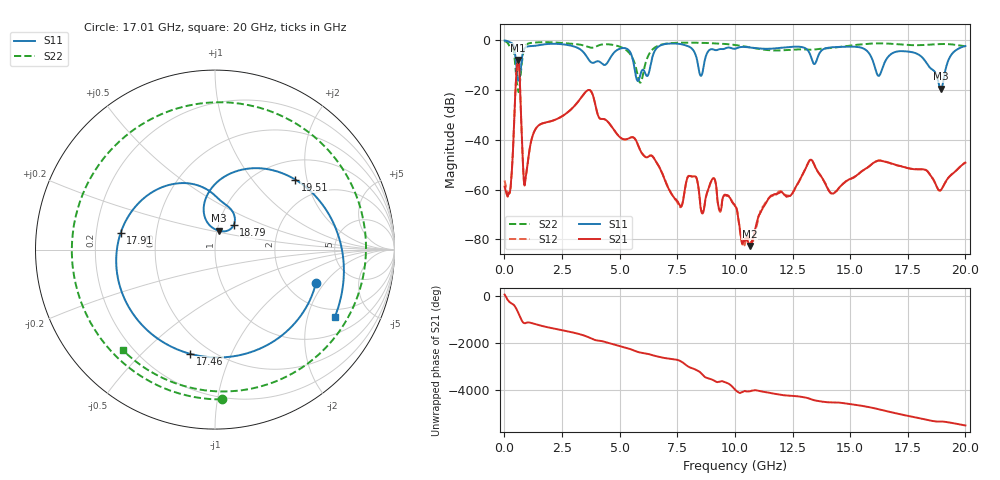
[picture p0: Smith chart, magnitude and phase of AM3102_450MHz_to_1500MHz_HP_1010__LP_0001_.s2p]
!Agilent Technologies,E8364B,MY43040894,A.07.50.67
!Agilent E8364B: A.07.50.67
!Date: Thursday, January 11, 2018 06:09:56
!Correction: S11(Full 2 Port(1,2))
!S21(Full 2 Port(1,2))
!S12(Full 2 Port(1,2))
!S22(Full 2 Port(1,2))
!S2P File: Measurements: S11, S21, S12, S22:
# Hz S  dB  R 50
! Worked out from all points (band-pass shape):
!   1601 points, 10 MHz to 20 GHz, reference 50 ohm
!   highest |S21| = -7.89 dB at 597.2 MHz (marker M1); lowest = -82.7 dB at 10.64 GHz (marker M2)
!   |S21| within 3 dB of the highest: 543 MHz to 644.9 MHz (101.9 MHz wide, 17.2 % of centre)
!   lowest |S11| = -19.4 dB at 18.94 GHz (marker M3), VSWR 1.24, Z = 51.1 + j10.8 ohm
!   |S11| at or under -10 dB: 5.621 GHz to 6.343 GHz (721.7 MHz wide, 12.1 % of centre); 16.05 GHz to 16.45 GHz (400.1 MHz wide, 2.46 % of centre); 18.38 GHz to 19.19 GHz (811.5 MHz wide, 4.32 % of centre)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
!   |S22| runs from -20.8 to -0.3 dB; largest |S21 - S12| = 0.0045
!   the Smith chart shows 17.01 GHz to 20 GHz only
!   S11 on the Smith chart (normalised r, x): 17.01 GHz: 2.86, -1.66; 17.46 GHz: 0.39, -0.71; 17.91 GHz: 0.31, +0.08; 18.79 GHz: 1.18, +0.33; 19.51 GHz: 1.42, +1.71; 20 GHz: 1.62, -2.97
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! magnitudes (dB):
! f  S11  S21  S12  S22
! 10 MHz  -0.1  -58.8  -56.3  -0.3
! 259.9 MHz  -0.9  -59.8  -60.0  -2.9
! 597.2 MHz  -15.8  -7.9  -7.9  -20.3
! 909.5 MHz  -2.9  -56.0  -56.0  -2.0
! 1.397 GHz  -2.1  -35.0  -35.0  -0.8
! 3.346 GHz  -4.0  -22.8  -22.8  -1.9
! 5.895 GHz  -14.0  -44.2  -44.2  -17.0
! 6.682 GHz  -2.5  -50.3  -50.3  -2.1
! 7.606 GHz  -1.5  -66.2  -66.7  -1.0
! 8.068 GHz  -2.8  -54.6  -54.5  -0.9
! 10.01 GHz  -3.4  -66.6  -66.1  -1.9
! 10.64 GHz  -2.9  -82.7  -80.4  -2.8
! 13.34 GHz  -7.8  -48.2  -48.2  -3.8
! 14.23 GHz  -2.8  -61.6  -61.5  -3.0
! 16.68 GHz  -6.3  -49.1  -49.2  -1.3
! 17.01 GHz  -4.5  -50.2  -50.2  -1.6
! 17.46 GHz  -4.5  -51.3  -51.3  -1.9
! 17.91 GHz  -5.5  -51.8  -51.8  -2.0
! 18.79 GHz  -15.3  -59.4  -59.4  -1.6
! 18.94 GHz  -19.4  -60.1  -60.2  -1.5
! 19.51 GHz  -4.5  -53.1  -53.0  -1.8
! 20 GHz  -2.3  -49.2  -49.0  -2.4
